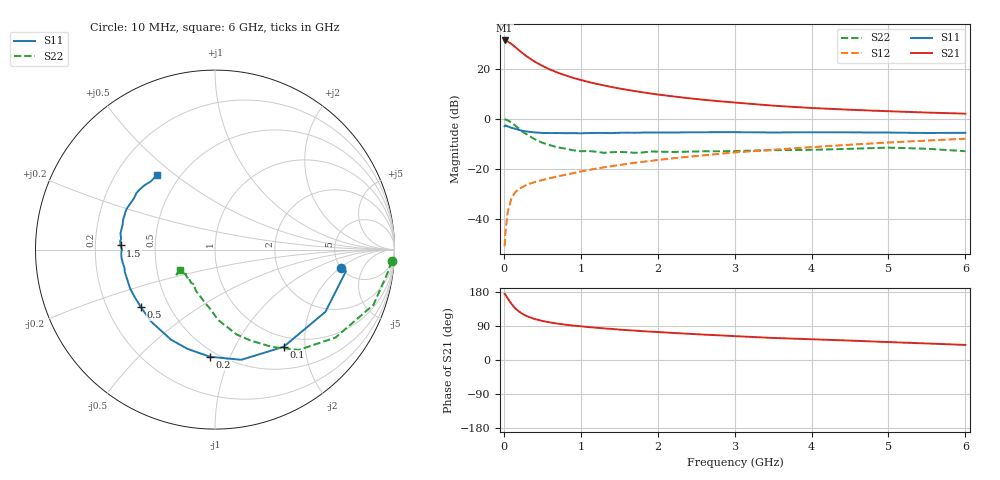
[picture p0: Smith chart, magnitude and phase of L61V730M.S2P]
!  INFINEON TECHNOLOGIES Small Signal Semiconductors
! BFR380L3 , Si-NPN RF-Transistor in TSLP-3-1
!  Vce=1.75 V,  Ic=30 mA
! Common Emitter S-Parameters:  07. March 2005
#  GHz  S  MA  R  50
! f  S11  S21  S12  S22
! GHz  Mag  Ang  Mag  Ang  Mag  Ang  Mag  Ang
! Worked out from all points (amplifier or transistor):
!   36 points, 10 MHz to 6 GHz, reference 50 ohm
!   highest |S21| = 31.2 dB at 10 MHz (marker M1)
!   |S21| within 3 dB of that: start of sweep to 162.8 MHz
!   unconditionally stable (mu >= 1): 1.812 GHz to 4.882 GHz
!   at 250 MHz: K = 0.40, MSG = 26.5 dB, |S12| = -27.1 dB
!   at 1.4 GHz: K = 0.97, MSG = 15.8 dB, |S12| = -18.9 dB
!   at 6 GHz: K = 0.98, MSG = 5.0 dB, |S12| = -7.9 dB
!   S11 on the Smith chart (normalised r, x): 10 MHz: 5.00, -2.13; 100 MHz: 0.83, -1.60; 200 MHz: 0.46, -0.85; 500 MHz: 0.35, -0.31; 1.5 GHz: 0.31, +0.02; 6 GHz: 0.38, +0.43
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0.01  0.7119 -8.5  36.39 174.6  0.0029 77.4  0.9869 -3.8
0.02  0.7393 -9.4  36.3 173.0  0.0053 85.1  0.9693 -7.9
0.05  0.7062 -29.4  34.75 162.5  0.0139 77.0  0.935 -19.2
0.1  0.6628 -54.8  30.88 147.8  0.0264 66.6  0.8314 -36.1
0.15  0.6312 -76.6  26.78 136.0  0.0348 58.9  0.7286 -50.1
0.2  0.5978 -92.6  23 127.4  0.0404 55.4  0.6298 -59.5
0.25  0.5739 -105.5  19.96 120.9  0.0444 52.9  0.5436 -68.7
0.3  0.5585 -116.0  17.4 115.7  0.0486 51.8  0.4888 -75.6
0.4  0.5362 -131.6  13.82 108.2  0.0548 51.1  0.3926 -87.4
0.5  0.523 -142.1  11.38 103.1  0.0603 51.9  0.3332 -94.4
0.6  0.5197 -150.1  9.58 99.1  0.0656 52.7  0.2975 -101.5
0.7  0.5202 -155.7  8.323 96.0  0.0714 54.8  0.2709 -108.2
0.8  0.5163 -161.5  7.339 93.2  0.0766 56.2  0.2543 -114.4
0.9  0.5179 -166.2  6.542 90.9  0.0823 57.7  0.2361 -119.1
1.1  0.5197 -172.2  5.421 86.9  0.0953 59.2  0.2282 -125.1
1.5  0.5267 177.5  4.028 80.2  0.1203 62.0  0.219 -135.0
1.8  0.5317 171.4  3.38 76.1  0.1387 62.6  0.2133 -140.5
2.2  0.533 165.1  2.796 71.4  0.1634 63.1  0.2184 -143.1
3.5  0.5341 147.7  1.829 58.2  0.2416 61.7  0.237 -147.8
4.5  0.5368 141.4  1.515 51.2  0.3046 60.1  0.2524 -147.2
5.5  0.5218 133.3  1.332 43.6  0.3686 56.4  0.253 -147.2
6  0.5264 128.1  1.266 39.8  0.4009 54.2  0.2265 -150.1
